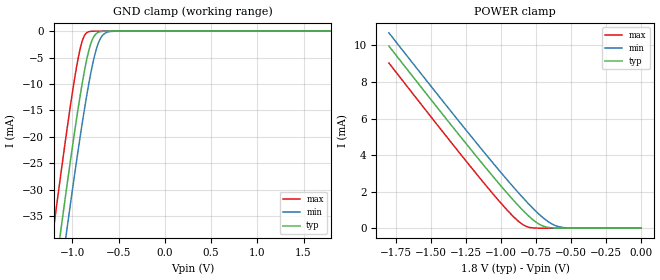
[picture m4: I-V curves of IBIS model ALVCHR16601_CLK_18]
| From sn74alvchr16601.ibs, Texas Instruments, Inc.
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[Model]   ALVCHR16601_CLK_18
Model_type  Input
Vinl=0.5775
Vinh=1.2675
| variable   typ   min   max
C_comp   1.91pF   1.72pF   2.15pF
[Temperature Range]   40   100   -40
| Ambient temperature   25   85   -40
[Voltage range]   1.8   1.65   1.95
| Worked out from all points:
|   GND clamp passes 1 mA (typ) near -0.77 V on its own axis
|   POWER clamp passes 1 mA (typ) near -0.85 V on its own axis
[GND Clamp]
| ALVCHR16601_CLK_18
|   Voltage   I(typ)   I(min)   I(max)
-1.8V     -129.9mA   -137.9mA   -119.8mA
-1.205V   -48.32mA   -56.61mA   -37.67mA
-1.125V   -37.81mA   -46.1mA    -27.15mA
-1.06V    -29.47mA   -37.73mA   -18.9mA
-980mV    -19.63mA   -27.72mA   -9.494mA
-925mV    -13.31mA   -21.13mA   -4.126mA
-880mV    -8.615mA   -16.01mA   -1.264mA
-835mV    -4.66mA    -11.26mA   -214.3uA
-780mV    -1.473mA   -6.233mA   -17.16uA
-725mV    -286.2uA   -2.598mA   -1.296uA
-615mV    -6.485uA   -167.9uA   -7.312nA
1.8V      3.326pA    6.145pA    3.026pA
[POWER Clamp]
| ALVCHR16601_CLK_18
|   Voltage   I(typ)   I(min)   I(max)
-1.8V     9.965mA    10.69mA    9.037mA
-1.38V    5.878mA    6.614mA    4.929mA
-1.105V   3.269mA    4.008mA    2.314mA
-940mV    1.776mA    2.501mA    856.4uA
-885mV    1.307mA    2.018mA    440uA
-845mV    982.9uA    1.676mA    200.1uA
-795mV    611.2uA    1.266mA    38.41uA
-715mV    166.7uA    670.1uA    941.7nA
-645mV    22.22uA    268.3uA    31.48nA
-585mV    2.717uA    77.14uA    1.709nA
-485mV    73.51nA    4.604uA    18.27pA
-16.28fV  3.324pA    5.122pA    3.398pA
